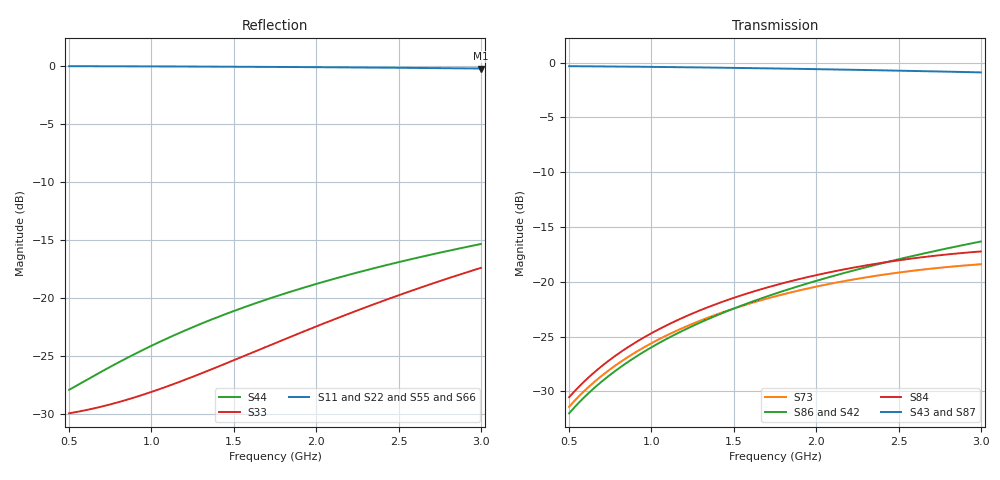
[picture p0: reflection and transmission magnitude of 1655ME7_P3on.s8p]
! Created Fri Dec 10 20:28:51 2010
# hz S db R 50
! 8 Port Network Data from SP1.SP block
! freq  dbS11  angS11  dbS12  angS12  dbS13  angS13  dbS14  angS14
!  dbS15  angS15  dbS16  angS16  dbS17  angS17  dbS18  angS18
!  dbS21  angS21  dbS22  angS22  dbS23  angS23  dbS24  angS24
!  dbS25  angS25  dbS26  angS26  dbS27  angS27  dbS28  angS28
!  dbS31  angS31  dbS32  angS32  dbS33  angS33  dbS34  angS34
!  dbS35  angS35  dbS36  angS36  dbS37  angS37  dbS38  angS38
!  dbS41  angS41  dbS42  angS42  dbS43  angS43  dbS44  angS44
!  dbS45  angS45  dbS46  angS46  dbS47  angS47  dbS48  angS48
!  dbS51  angS51  dbS52  angS52  dbS53  angS53  dbS54  angS54
!  dbS55  angS55  dbS56  angS56  dbS57  angS57  dbS58  angS58
!  dbS61  angS61  dbS62  angS62  dbS63  angS63  dbS64  angS64
!  dbS65  angS65  dbS66  angS66  dbS67  angS67  dbS68  angS68
!  dbS71  angS71  dbS72  angS72  dbS73  angS73  dbS74  angS74
!  dbS75  angS75  dbS76  angS76  dbS77  angS77  dbS78  angS78
!  dbS81  angS81  dbS82  angS82  dbS83  angS83  dbS84  angS84
!  dbS85  angS85  dbS86  angS86  dbS87  angS87  dbS88  angS88
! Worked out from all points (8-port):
!   251 points, 500 MHz to 3 GHz, reference 50 ohm
!   strongest paths, dB at 500 MHz, 1.12 GHz, 1.75 GHz, 2.38 GHz, 3 GHz:
!     S43: -0.3, -0.4, -0.5, -0.7, -0.9
!     S87: -0.3, -0.4, -0.5, -0.7, -0.9
!     S84: -30.5, -23.8, -20.3, -18.3, -17.2
!     S86: -32.0, -25.0, -21.1, -18.4, -16.3
!     S42: -32.1, -25.1, -21.2, -18.6, -16.5
!     S73: -31.4, -24.7, -21.3, -19.4, -18.4
!   lowest |S11| = -0.2 dB at 3 GHz (marker M1), VSWR 75.25, Z = 21.9 - j282 ohm
!   |S11| at or under -10 dB: nowhere
